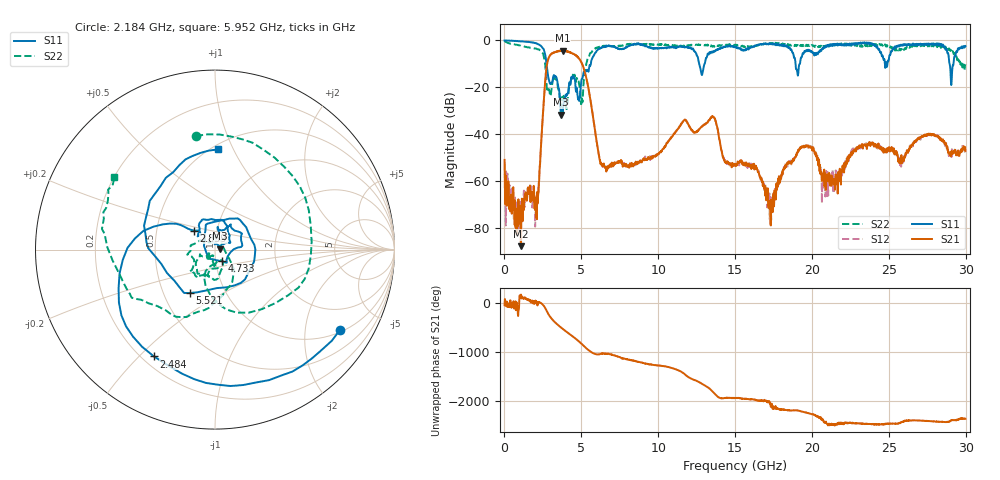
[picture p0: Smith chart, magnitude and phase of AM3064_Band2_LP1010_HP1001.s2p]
# Hz S DB R 50.0
!freq dBS11 angS11 dBS21 angS21 dBS12 angS12 dBS22 angS22
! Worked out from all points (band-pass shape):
!   1600 points, 10 MHz to 29.98 GHz, reference 50 ohm
!   highest |S21| = -4.42 dB at 3.777 GHz (marker M1); lowest = -87.7 dB at 1.078 GHz (marker M2)
!   |S21| within 3 dB of the highest: 2.88 GHz to 4.817 GHz (1.937 GHz wide, 50.3 % of centre)
!   lowest |S11| = -31.7 dB at 3.665 GHz (marker M3), VSWR 1.05, Z = 52.6 + j0.481 ohm
!   |S11| at or under -10 dB: 2.732 GHz to 5.619 GHz (2.887 GHz wide, 69.1 % of centre); 12.67 GHz to 13.02 GHz (354.9 MHz wide, 2.76 % of centre); 18.93 GHz to 19.22 GHz (284.9 MHz wide, 1.49 % of centre)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
!   |S22| runs from -29.2 to -0.3 dB; largest |S21 - S12| = 0.016
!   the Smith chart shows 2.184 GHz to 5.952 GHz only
!   S11 on the Smith chart (normalised r, x): 2.184 GHz: 1.08, -3.07; 2.484 GHz: 0.25, -0.55; 2.859 GHz: 0.77, +0.17; 4.733 GHz: 1.08, -0.14; 5.521 GHz: 0.68, -0.36; 5.952 GHz: 0.54, +0.87
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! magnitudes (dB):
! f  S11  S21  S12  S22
! 10 MHz  0.0  -50.9  -52.4  -0.3
! 1.078 GHz  -0.4  -87.7  -70.6  -2.4
! 2.184 GHz  -1.6  -66.4  -62.0  -3.8
! 2.484 GHz  -3.3  -33.2  -33.3  -5.5
! 2.859 GHz  -16.0  -7.8  -7.8  -21.0
! 3.665 GHz  -31.7  -4.6  -4.4  -26.3
! 3.777 GHz  -30.6  -4.4  -4.4  -26.5
! 4.733 GHz  -22.3  -6.8  -6.9  -16.6
! 5.015 GHz  -16.6  -9.5  -9.6  -25.0
! 5.521 GHz  -11.1  -22.5  -22.5  -6.4
! 5.952 GHz  -5.1  -41.0  -41.1  -3.2
! 6.645 GHz  -2.3  -54.5  -55.4  -2.5
! 10 GHz  -3.4  -48.3  -48.1  -1.8
! 13.54 GHz  -5.2  -32.5  -32.4  -2.6
! 15 GHz  -2.7  -53.3  -52.6  -1.9
! 16.37 GHz  -2.1  -54.7  -54.7  -2.4
! 17.31 GHz  -1.7  -78.6  -79.1  -1.4
! 19.99 GHz  -4.8  -45.8  -45.8  -2.0
! 20.8 GHz  -2.7  -55.1  -59.3  -2.5
! 25 GHz  -8.5  -45.7  -47.1  -2.2
! 29.08 GHz  -17.8  -47.1  -49.7  -5.0
! 29.98 GHz  -2.4  -47.0  -46.1  -10.2
